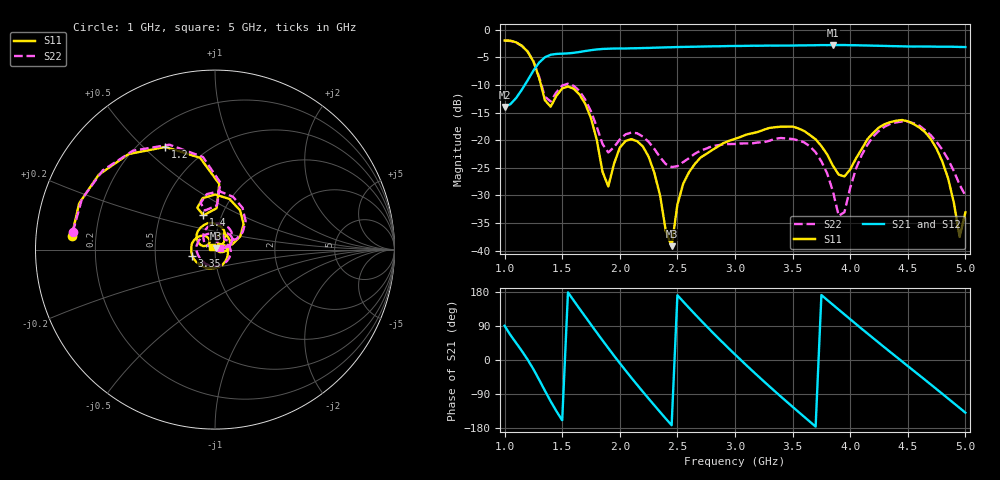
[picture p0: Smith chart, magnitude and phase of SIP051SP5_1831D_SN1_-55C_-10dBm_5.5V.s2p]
# GHz  S  dB  R  50
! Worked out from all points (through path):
!   81 points, 1 GHz to 5 GHz, reference 50 ohm
!   highest |S21| = -2.74 dB at 3.85 GHz (marker M1); lowest = -14.0 dB at 1 GHz (marker M2)
!   lowest |S11| = -39.2 dB at 2.45 GHz (marker M3), VSWR 1.02, Z = 50.7 + j0.867 ohm
!   |S11| at or under -10 dB: 1.316 GHz to end of sweep
!   |S22| runs from -33.7 to -2.0 dB; largest |S21 - S12| = 0.0029
!   S11 on the Smith chart (normalised r, x): 1 GHz: 0.11, +0.05; 1.2 GHz: 0.30, +0.58; 1.4 GHz: 0.82, +0.33; 3.35 GHz: 0.77, -0.05; 5 GHz: 0.97, +0.03
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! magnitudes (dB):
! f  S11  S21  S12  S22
! 1 GHz  -1.9  -14.0  -14.0  -2.0
! 1.2 GHz  -3.9  -9.1  -9.1  -3.9
! 1.4 GHz  -13.9  -4.5  -4.5  -13.0
! 1.55 GHz  -10.3  -4.3  -4.3  -9.7
! 1.7 GHz  -13.4  -3.8  -3.8  -12.7
! 1.9 GHz  -28.4  -3.4  -3.4  -22.2
! 2.1 GHz  -19.8  -3.3  -3.3  -18.6
! 2.35 GHz  -30.0  -3.2  -3.2  -23.1
! 2.45 GHz  -39.2  -3.1  -3.1  -24.9
! 2.5 GHz  -31.7  -3.1  -3.1  -24.7
! 2.6 GHz  -25.8  -3.1  -3.1  -23.3
! 3 GHz  -19.7  -2.9  -2.9  -20.7
! 3.35 GHz  -17.6  -2.9  -2.9  -19.7
! 3.7 GHz  -19.8  -2.8  -2.8  -22.2
! 3.85 GHz  -24.6  -2.7  -2.7  -29.3
! 3.95 GHz  -26.6  -2.7  -2.7  -33.0
! 4.1 GHz  -21.6  -2.8  -2.8  -22.7
! 4.35 GHz  -16.7  -2.9  -3.0  -17.0
! 4.7 GHz  -19.8  -3.0  -3.0  -19.1
! 4.85 GHz  -26.9  -3.0  -3.1  -23.5
! 4.95 GHz  -37.5  -3.1  -3.1  -28.1
! 5 GHz  -33.1  -3.1  -3.1  -30.0
